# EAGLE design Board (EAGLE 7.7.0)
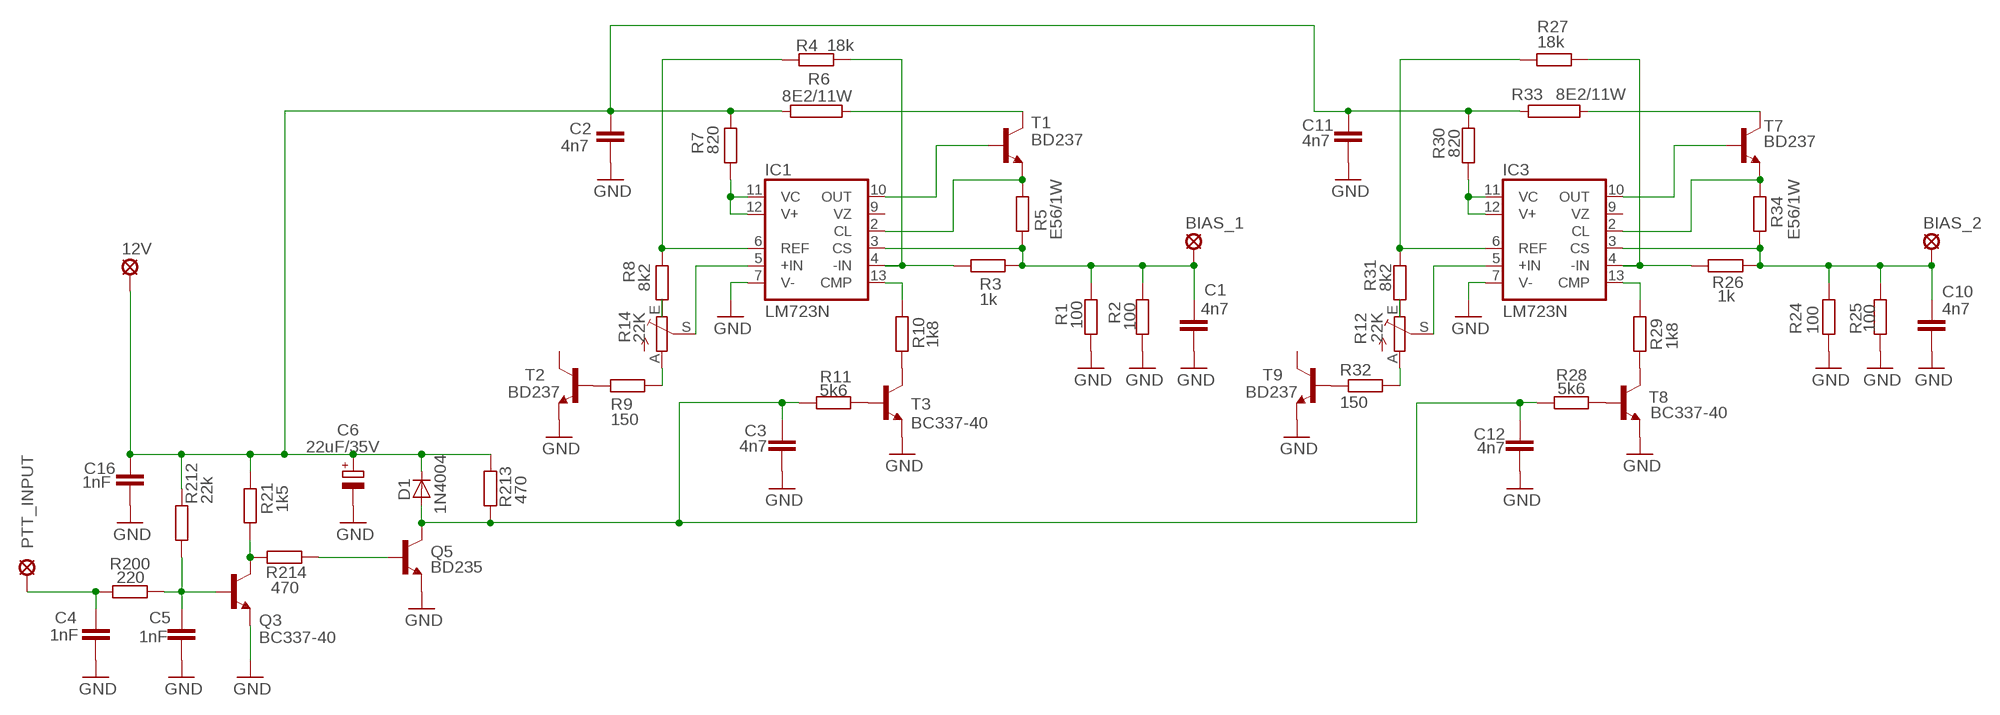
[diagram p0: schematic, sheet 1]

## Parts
12V  MCS10B  [MCS10B]
BIAS_1  MCS10B  [MCS10B]
BIAS_2  MCS10B  [MCS10B]
C1  4n7  C-EU050-024X044  [C050-024X044]
C2  4n7  C-EU050-024X044  [C050-024X044]
C3  4n7  C-EU050-024X044  [C050-024X044]
C4  1nF  C-EU050-024X044  [C050-024X044]
C5  1nF  C-EU050-024X044  [C050-024X044]
C6  22uF/35V  CPOL-EUE5-8.5  [E5-8,5]
C10  4n7  C-EU050-024X044  [C050-024X044]
C11  4n7  C-EU050-024X044  [C050-024X044]
C12  4n7  C-EU050-024X044  [C050-024X044]
C16  1nF  C-EU050-024X044  [C050-024X044]
D1  1N4004  [DO41-10]
IC1  LM723N  [DIL14]
IC3  LM723N  [DIL14]
PTT_INPUT  MCS10B  [MCS10B]
Q3  BC337-40  [TO92]
Q5  BD235  [TO126]
R1  100  R-EU_0207/10  [0207/10]
R2  100  R-EU_0207/10  [0207/10]
R3  1k  R-EU_0207/10  [0207/10]
R4  18k  R-EU_0207/10  [0207/10]
R5  E56/1W  R-EU_0613/15  [P0613/15]
R6  8E2/11W  RKH216-8  [KH216-8]
R7  820  R-EU_0207/10  [0207/10]
R8  8k2  R-EU_0207/10  [0207/10]
R9  150  R-EU_0207/10  [0207/10]
R10  1k8  R-EU_0207/10  [0207/10]
R11  5k6  R-EU_0207/10  [0207/10]
R12  22K  TRIM_EU-B64W  [B64W]
R14  22K  TRIM_EU-B64W  [B64W]
R21  1k5  R-EU_0207/10  [0207/10]
R24  100  R-EU_0207/10  [0207/10]
R25  100  R-EU_0207/10  [0207/10]
R26  1k  R-EU_0207/10  [0207/10]
R27  18k  R-EU_0207/10  [0207/10]
R28  5k6  R-EU_0207/10  [0207/10]
R29  1k8  R-EU_0207/10  [0207/10]
R30  820  R-EU_0207/10  [0207/10]
R31  8k2  R-EU_0207/10  [0207/10]
R32  150  R-EU_0207/10  [0207/10]
R33  8E2/11W  RKH216-8  [KH216-8]
R34  E56/1W  R-EU_0613/15  [P0613/15]
R200  220  R-EU_0207/10  [0207/10]
R212  22k  R-EU_0207/10  [0207/10]
R213  470  R-EU_0207/10  [0207/10]
R214  470  R-EU_0207/10  [0207/10]
T1  BD237  BD235  [TO126]
T2  BD237  BD235  [TO126]
T3  BC337-40  [TO92]
T7  BD237  BD235  [TO126]
T8  BC337-40  [TO92]
T9  BD237  BD235  [TO126]

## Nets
N$1: R29.2 T8.3(C)
N$2: IC1.13(CMP) R10.1
N$3: C3.1 C12.1 D1.A Q5.2(C) R11.1 R28.1 R213.1
N$4: R11.2 T3.2(B)
N$5: IC1.11(VC) IC1.12(V+) R7.1
N$6: C4.1 PTT_INPUT.MP R200.1
N$7: R6.2 T1.2(C)
N$8: IC1.10(OUT) T1.3(B)
N$9: IC1.2(CL) R5.2 T1.1(E)
N$10: BIAS_1.MP C1.1 IC1.3(CS) R1.2 R2.2 R3.2 R5.1
N$11: IC1.4(-IN) R3.1 R4.2
N$12: IC1.5(+IN) R14.S
N$13: IC1.6(REF) R4.1 R8.2
N$14: R8.1 R14.E
N$15: R9.2 R14.A
N$16: R9.1 T2.3(B)
N$17: C1.2 C2.2 C3.2 C4.2 C5.2 C6.- C10.2 C11.2 C12.2 C16.2 IC1.7(V-) IC3.7(V-) Q3.1(E) Q5.1(E) R1.1 R2.1 R24.1 R25.1 T2.1(E) T3.1(E) T8.1(E) T9.1(E) ; supply symbol labelled GND
N$18: 12V.MP C2.1 C6.+ C11.1 C16.1 D1.C R6.1 R7.2 R21.2 R30.2 R33.1 R212.2 R213.2
N$20: R10.2 T3.3(C)
N$22: C5.1 Q3.2(B) R200.2 R212.1
N$34: IC3.13(CMP) R29.1
N$35: R28.2 T8.2(B)
N$37: IC3.11(VC) IC3.12(V+) R30.1
N$38: Q3.3(C) R21.1 R214.1
N$39: R33.2 T7.2(C)
N$40: IC3.10(OUT) T7.3(B)
N$41: IC3.2(CL) R34.2 T7.1(E)
N$42: BIAS_2.MP C10.1 IC3.3(CS) R24.2 R25.2 R26.2 R34.1
N$43: IC3.4(-IN) R26.1 R27.2
N$44: IC3.5(+IN) R12.S
N$45: IC3.6(REF) R27.1 R31.2
N$46: R12.E R31.1
N$47: R12.A R32.2
N$48: R32.1 T9.3(B)
N$54: Q5.3(B) R214.2
Unconnected: IC1.9(VZ) IC3.9(VZ) T2.2(C) T9.2(C)

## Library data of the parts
12V BIAS_1 BIAS_2 PTT_INPUT = solpad:MCS10B: SOLDER PAD
C1-C5 C10-C12 C16 = rcl:C-EU: CAPACITOR, European symbol
C6 = rcl:CPOL-EU: POLARIZED CAPACITOR, European symbol
D1 = diode:1N4004: DIODE
IC1 IC3 = linear:*723: Positive VOLTAGE REGULATOR
Q3 T3 T8 = transistor-npn:BC337*: NPN Transistor
Q5 T1 T2 T7 T9 = transistor-npn:BD235*: NPN Transistor
R1-R5 R7-R11 R21 R24-R32 R34 R200 R212-R214 = rcl:R-EU_: RESISTOR, European symbol
R6 R33 = resistor-power:R: Power Resitor
R12 R14 = pot:TRIM_EU-: POTENTIOMETER

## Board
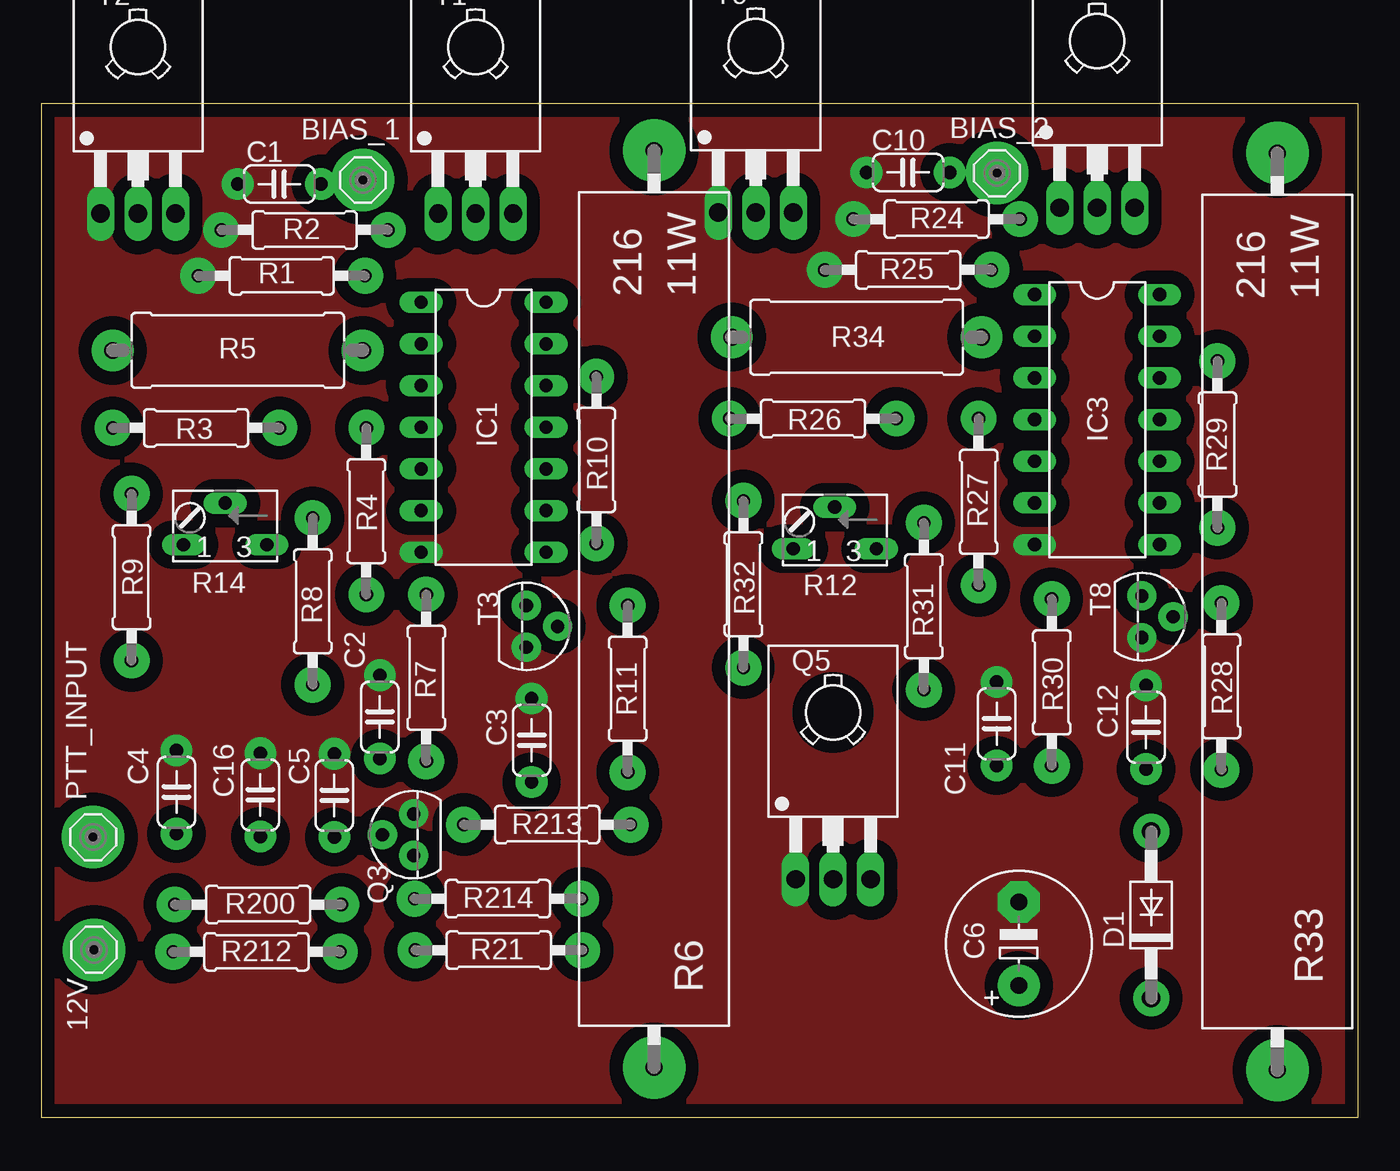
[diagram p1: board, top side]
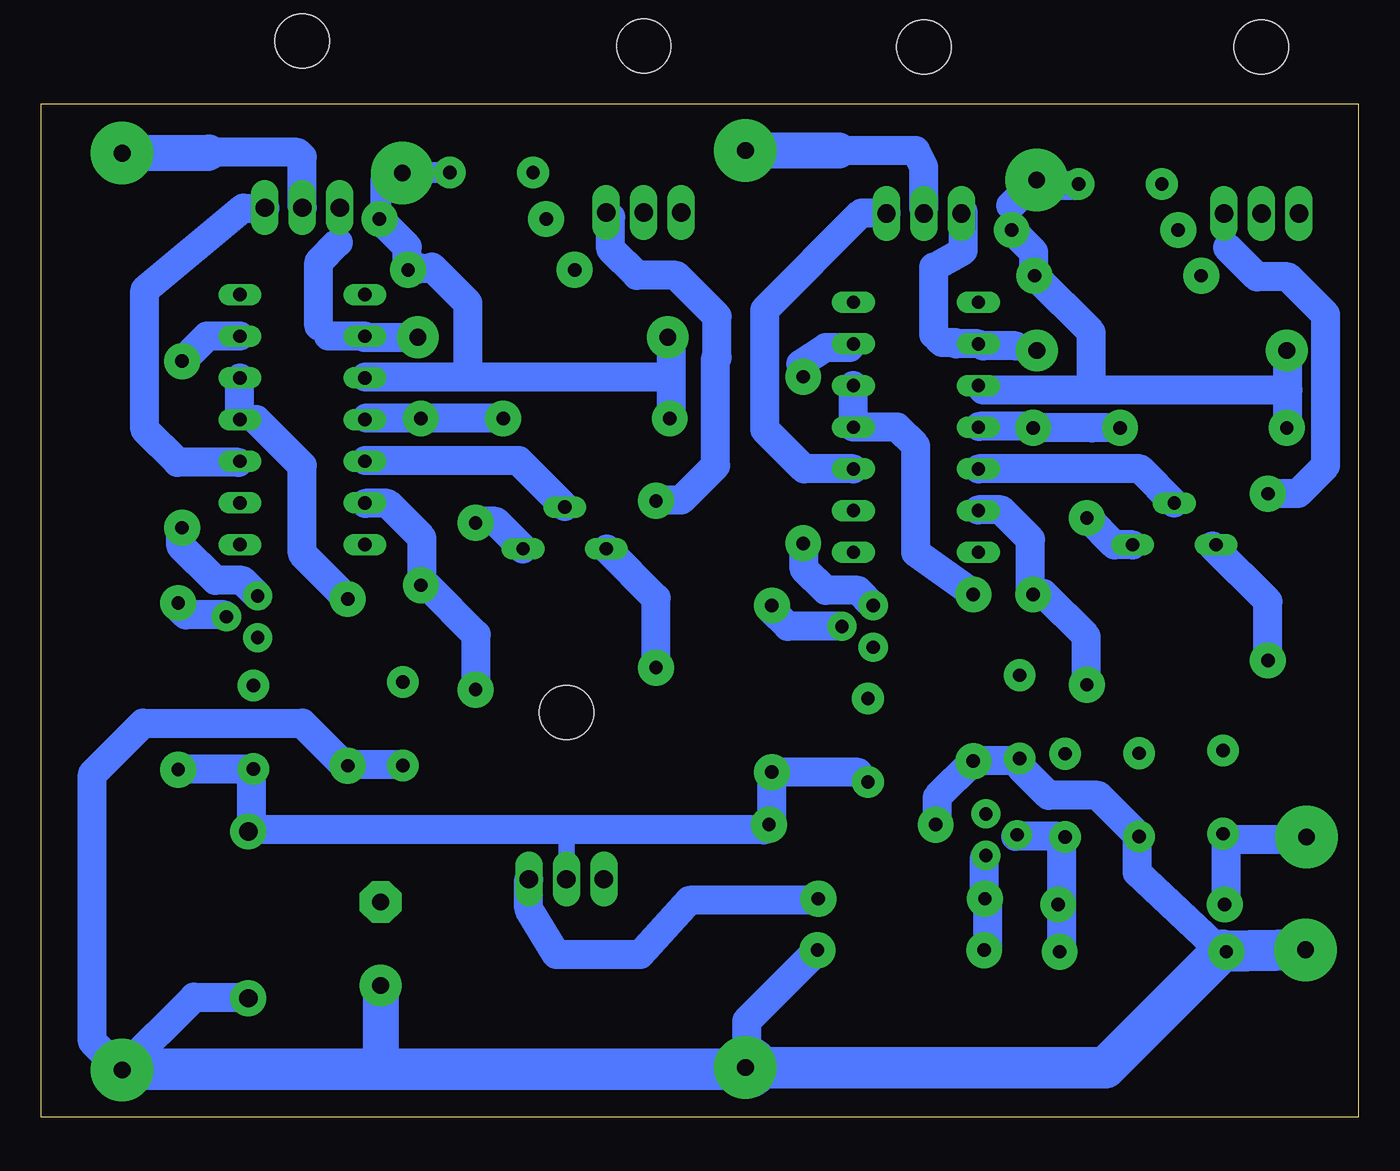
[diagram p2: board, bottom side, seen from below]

Size 80.33 x 61.8 mm. Coordinates in mm from the lower left corner, seen from the top.
Outline: 0,0 80.33,0 80.33,61.8 0,61.8 0,0
Copper layers (1*16): Top 0.035mm / dielectric 1.5mm / Bottom 0.035mm
Design rules "default": minimum track width 10mil, minimum drill 24mil, track to track 8mil, track to pad 8mil, pad to pad 8mil, via to via 8mil, smd to smd 8mil, copper to edge 20mil, drill to drill 8mil, minimum pad ring 10mil, minimum via ring 8mil, stop-mask expansion 4mil, vias tented up to drill 0mil, thermal gap 10mil

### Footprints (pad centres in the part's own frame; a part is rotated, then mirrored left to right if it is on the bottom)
MCS10B = drill 1.016 pad 3.81: MP 0,0
C050-024X044 = drill 0.813 pad 1.93: 1 -2.54,0; 2 2.54,0
E5-8,5 = drill 1.016 pad 2.54: + -2.54,0 | drill 1.016 pad 2.54 octagon: - 2.54,0
DO41-10 = drill 1.118 pad 2.184: A 5.08,0; C -5.08,0
DIL14 = drill 0.813 long: 1 -7.62,-3.81; 2 -5.08,-3.81; 3 -2.54,-3.81; 4 0,-3.81; 5 2.54,-3.81; 6 5.08,-3.81; 7 7.62,-3.81; 8 7.62,3.81; 9 5.08,3.81; 10 2.54,3.81; 11 0,3.81; 12 -2.54,3.81; 13 -5.08,3.81; 14 -7.62,3.81
TO92 = drill 0.813 pad 1.778: 1 1.27,0; 2 0,1.905; 3 -1.27,0
TO126 = drill 1.118 long: 1 -2.286,-5.08; 2 0,-5.08; 3 2.286,-5.08 | hole 3.302: 0,5.08
0207/10 = drill 0.813 pad 2.184: 1 -5.08,0; 2 5.08,0
P0613/15 = drill 1.016 pad 2.54: 1 -7.62,0; 2 7.62,0
KH216-8 = drill 1.016 pad 3.81: 1 -27.94,0; 2 27.94,0
B64W = drill 0.813 long: A 2.54,0; E -2.54,0; S 0,-2.54

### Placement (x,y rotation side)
12V  3.23,10.22 0 top
BIAS_1  19.63,57.14 0 top
BIAS_2  58.29,57.56 0 top
C1  14.53,56.89 180 top
C2  20.66,24.41 90 top
C3  29.91,22.99 90 top
C4  8.26,19.83 90 top
C5  17.88,19.63 90 top
C6  59.62,10.59 90 top
C10  52.87,57.6 180 top
C11  58.27,24 90 top
C12  67.37,23.78 90 top
C16  13.37,19.66 90 top
D1  67.69,12.35 90 top
IC1  26.99,42.07 270 top
IC3  64.4,42.54 270 top
PTT_INPUT  3.18,17.09 0 top
Q3  22.71,17.24 90 top
Q5  48.29,19.6 0 top
R1  14.67,51.3 0 top
R2  16.07,54.1 0 top
R3  9.45,42.03 180 top
R4  19.83,36.95 90 top
R5  11.99,46.75 0 top
R6  37.38,30.99 90 top
R7  23.49,26.8 270 top
R8  16.56,31.46 270 top
R9  5.52,32.94 270 top
R10  33.86,40.07 270 top
R11  35.77,26.13 90 top
R12  48.4,34.66 180 top
R14  11.23,34.9 180 top
R21  27.91,10.2 0 top
R24  54.61,54.76 0 top
R25  52.87,51.66 0 top
R26  47.07,42.6 180 top
R27  57.17,37.52 90 top
R28  71.97,26.28 90 top
R29  71.73,41.02 270 top
R30  61.63,26.52 270 top
R31  53.83,31.16 270 top
R32  42.83,32.5 270 top
R33  75.38,30.83 90 top
R34  49.73,47.56 0 top
R200  13.24,12.98 0 top
R212  13.14,10.1 180 top
R213  30.86,17.85 180 top
R214  27.86,13.33 0 top
T1  26.49,60.17 0 top
T2  5.92,60.17 0 top
T3  29.59,29.93 270 top
T7  64.4,60.53 0 top
T8  67.12,30.52 270 top
T9  43.58,60.23 0 top

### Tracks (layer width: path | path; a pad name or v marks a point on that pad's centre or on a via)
N$1
  Bottom 1.016: 71.8,35.87 R29.2
  Bottom 1.778: T8.3 68.06,32.73 69.7,32.73 71.8,34.83 71.8,35.87
N$2
  Bottom 1.27: IC1.13 31.02,46.93 | R10.1 33.58,45.43 34,45.43 34,45.93
  Bottom 1.778: 31.02,46.93 32.5,46.93 34,45.93
N$3
  Bottom 0.406: R28.1 71.93,21.2 71.89,21.24
  Bottom 1.016: D1.A 67.7,17.53 67.5,17.73 | 36.27,17.53 R213.1 35.82,17.73 35.8,17.73 | Q5.2 48.3,17.53 | 35.8,21.03 35.79,21.03 R11.1 35.8,21.02 | C3.1 30.49,21.03
  Bottom 1.27: 67.5,21.24 C12.1
  Bottom 1.778: 71.89,21.24 67.5,21.24 67.5,17.73 | 36.27,17.53 48.3,17.53 67.7,17.53 | 30.49,21.03 35.79,21.03 | 35.8,21.02 35.8,17.73
N$4
  Bottom 1.016: T3.2 | 35.8,31.24 35.8,31.33 | 35.8,31.24 R11.2 | 35.8,30.93 35.8,31.24
  Bottom 1.778: T3.2 34.8,29.93 35.8,30.93
N$5
  Bottom 0.406: IC1.11 30.8,42.13 30.5,42.43 30.8,42.73 | R7.1 23.49,31.92
  Bottom 1.778: 30.8,42.73 IC1.12 | IC1.11 28.14,42.07 27,40.93 27,34.43 23.49,31.92
N$6
  Bottom 0.61: 3.34,16.93 PTT_INPUT.MP | 8.1,12.93 8.1,13.12 R200.1 | 8.1,16.93 C4.1
  Bottom 1.778: 3.34,16.93 8.1,16.93 8.1,13.12
N$7
  Bottom 0.406: 26.5,55.43 26.49,55.43 T1.2
  Bottom 1.778: 26.5,55.43 26.5,57.93 27,58.93 31.7,58.93
  Bottom 1.93: 31.7,58.93 32,58.93
  Bottom 2.184: R6.2 31.7,58.93
N$8
  Bottom 1.016: IC1.10 | 28.8,55.13 28.8,55.11 T1.3
  Bottom 1.778: IC1.10 33.8,39.53 36.2,41.93 36.2,49.23 30.3,55.13 28.8,55.13
N$9
  Bottom 1.016: IC1.2 23.1,47.23 22.9,47.03 | 20.7,47.03 20.9,47.03 19.89,47.03 R5.2 | 24.52,47.15 24.6,47.23 | 24.1,55.23 24.1,55.2 T1.1
  Bottom 1.778: 20.9,47.03 22.9,47.03 | IC1.2 24.52,47.15 | 24.6,47.23 25.4,47.23 25.9,47.73 25.9,51.83 24.1,52.83 24.1,55.2
N$10
  Bottom 1.016: BIAS_1.MP 19.61,57.13 19.4,57.13 19.1,56.83 | 17.1,56.83 17.1,56.86 C1.1 | R2.2 21.2,54.14 21.2,55.57 | 4.3,46.73 4.35,46.73 R5.1 | R3.2 4.3,42.11 | 22.89,44.33 IC1.3 | 19.8,51.33 19.78,51.33 R1.2
  Bottom 1.778: 19.1,56.83 17.1,56.83 | 21.2,55.57 BIAS_1.MP | 4.3,42.11 4.3,44.33 | 4.3,44.33 4.3,46.73 | 4.3,44.33 16.3,44.33 | 16.3,44.33 22.89,44.33 | R2.2 19.8,52.74 19.8,51.33 | R1.2 16.3,47.85 16.3,44.33
N$11
  Bottom 1.016: R4.2 19.93,42.13 | 23.12,42.13 IC1.4
  Bottom 1.778: R3.1 16.24,42.03 R4.2 | 19.93,42.13 23.12,42.13
N$12
  Bottom 1.016: IC1.5
  Bottom 1.778: R14.S 13.32,39.53 IC1.5
N$13
  Bottom 1.016: R8.2 16.6,26.42 | 19.2,31.93 19.8,31.93 19.8,31.91 R4.1 20,32.04 | 23.2,37.03 23.2,37.01 IC1.6
  Bottom 1.778: 16.6,26.42 16.6,29.33 19.2,31.93 | 20,32.04 20,35.23 21.8,37.03 23.2,37.03
N$14
  Bottom 0.406: R8.1 16.66,37.09
  Bottom 1.016: 16.51,36.54 R8.1
  Bottom 1.778: R14.E 14.87,34.9 16.51,36.54
N$15
  Bottom 1.27: 8.9,34.83 8.82,34.9 R14.A
  Bottom 1.778: R9.2 5.52,31.46 8.9,34.83
N$16
  Bottom 1.016: 5.51,38.03 R9.1 | T2.3 8,54.88 8,53.03
  Bottom 1.778: 5.51,38.03 3.7,38.03 2,39.73 2,48.93 4.3,51.23 6.2,51.23 8,53.03
N$17
  pour Top (isolate 0.813, no thermals): 0.3,61.13 0.3,0.23 79.7,0.23 79.7,61.33
N$18
  Bottom 0.406: 8.4,10.13 10.19,7.33 R212.2
  Bottom 0.61: 8.46,10.13 R212.2 | 12V.MP 3.24,10.23
  Bottom 1.016: 58.34,21.53 C11.1 | 61.9,21.53 61.7,21.33 | 75.4,2.93 75.4,2.91 R33.1 75.4,2.87 | 75.4,2.93 75.5,2.93 | 37.3,2.93 37.3,3.05 | 67.75,7.33 D1.C | 75.4,2.87 75.4,2.83 | 75.4,2.93 75.4,2.87 | 59.6,2.93 59.6,2.53 | 59.6,8.03 C6.+
  Bottom 1.27: 13.5,16.75 C16.1 | R30.2 61.51,21.44 61.5,21.43 61.47,21.46 C11.1
  Bottom 1.778: 13.5,16.75 13.5,14.93 8.4,10.13 | 58.34,21.53 61.9,21.53 64.4,24.03 74.1,24.03 77.2,20.93 77.2,4.63 75.5,2.93 | 67.75,7.33 71,7.33 75.4,2.93 | R21.2 37.3,5.89 37.3,4.63 | 37.3,4.63 37.3,3.73 | C16.1 15.88,19.63 18.9,19.63 20.6,21.33 20.6,21.93 C2.1 20.8,21.73 R7.2 | R7.2 | R7.2 25.7,19.51 25.7,17.93 25.71,17.93 R213.2 | R6.1 37.3,3.13 37.3,4.63
  Bottom 1.93: R212.2 8.27,10.2
  Bottom 2.184: 59.6,2.93 59.6,8.03
  Bottom 2.54: 3.24,10.23 8.46,10.13 | 37.5,2.93 37.3,2.93 | 37.5,2.93 59.6,2.93 75.4,2.93 | 37.5,2.93 37.5,3.03 15.44,3.03 8.27,10.2
  Bottom 3.81: 37.3,3.05 R6.1
N$20
  Bottom 1.016: 33.8,35.03 33.82,35.03 R10.2
  Bottom 1.778: T3.3 30.52,32.13 32.5,32.13 33.8,33.43 33.8,35.03
N$22
  Bottom 0.406: 21,17.13 20.92,17.13 Q3.2 | 18.1,17.03 18.3,17.13 | 18.6,13.43 18.57,13.43 R200.2 | 18.1,13.23 18.6,13.43 | 18.6,13.43 18.8,13.43
  Bottom 0.61: R212.1 18.1,10.52 | 18.1,17.03 18.04,16.93 C5.1
  Bottom 1.778: 18.1,10.52 18.1,13.23 18.1,17.03 | 18.3,17.13 20.92,17.13
N$34
  Bottom 1.778: IC3.13 70.21,47.62 R29.1
N$35
  Bottom 1.016: T8.2 69.13,30.63 | R28.2 72,31.33 72,31.13
  Bottom 1.778: 69.13,30.63 71.5,30.63 72,31.13
N$37
  Bottom 0.406: IC3.11 68.21,42.62 68.1,42.73 68.15,42.78 68.21,42.84
  Bottom 1.016: 68.15,42.78 68.4,42.53 67.2,42.53
  Bottom 1.778: 68.21,42.84 IC3.12 | R30.1 64.4,34.37 64.4,39.73 67.2,42.53
N$38
  Bottom 0.406: 22.8,13.23 22.8,13.31 R214.1 22.6,13.16 | 22.8,15.88 Q3.3 | R21.1 22.6,10.43
  Bottom 1.778: 22.8,13.31 22.8,15.88 | 22.6,10.43 22.6,13.16
N$39
  Bottom 1.778: T7.2 64.4,58.53 64.7,58.83 70.1,58.83 70.2,58.73 70.2,58.77
  Bottom 2.184: R33.2 70.2,58.77 70.16,58.77 70.1,58.83
N$40
  Bottom 0.406: T7.3
  Bottom 1.27: IC3.10 68.28,39.93 | 66.5,55.43 66.66,55.43 T7.3
  Bottom 1.778: 68.28,39.93 72,39.93 74,41.93 74,50.43 68,55.43 66.66,55.43
N$41
  Bottom 1.016: 60.6,47.53 IC3.2 | R34.2 57.38,47.53 | 62.8,47.63 63.4,48.23 | T7.1 62.2,55.36 62.2,53.33
  Bottom 1.778: 57.38,47.53 60.6,47.53 | IC3.2 62.8,47.63 | 63.4,48.23 63.4,52.13 62.2,53.33
N$42
  Bottom 0.406: 59.6,57.13 59.15,57.58 59.13,57.6 | 59.69,54.84 59.7,54.83 | R24.2 59.69,54.84 | 59.69,54.84 59.6,54.93
  Bottom 1.016: R26.2 41.9,42.69 | 41.9,47.35 R34.1 | 60.54,45.13 IC3.3 | 57.6,51.71 R25.2 57.38,51.83 | 54.3,45.13 54.3,45.03 | 59.15,57.58 59.2,57.63 58.36,57.63 BIAS_2.MP
  Bottom 1.27: 59.13,57.6 C10.1 | 59.6,54.93 59.6,57.13
  Bottom 1.778: 41.9,42.69 41.9,45.13 | 41.9,45.13 41.9,47.35 | 41.9,45.13 54.3,45.13 | 54.3,45.13 60.54,45.13 | 54.3,45.13 54.3,49.63 56.5,51.83 56.6,51.73 57.28,51.73 57.38,51.83 | R25.2 58,51.71 58,53.07 R24.2
N$43
  Bottom 1.016: 57.2,42.63 57.3,42.63 | 57.2,42.63 R27.2 | R26.1 52.18,42.63 | 56.9,42.63 57.2,42.63 | 60.5,42.63 IC3.4
  Bottom 1.778: 52.18,42.63 56.9,42.63 60.5,42.63
N$44
  Bottom 1.016: 60.56,40.03 IC3.5 | 48.3,37.23 48.37,37.23 | 48.37,37.23 R12.S | 48.37,37.23 48.4,37.23
  Bottom 1.778: 60.56,40.03 51.2,40.03 48.4,37.23
N$45
  Bottom 1.016: R31.2 53.8,26.11 | 56.8,32.43 R27.1 57.1,32.51 | 60.56,37.43 IC3.6
  Bottom 1.778: 53.8,26.11 53.8,29.43 56.8,32.43 | 57.1,32.51 57.1,35.33 59.2,37.43 60.56,37.43
N$46
  Bottom 1.016: 53.8,36.33 53.8,36.27 R31.1
  Bottom 1.778: R12.E 52.61,36.33 53.8,36.33
N$47
  Bottom 0.406: 45.83,34.66 R12.A
  Bottom 1.778: R32.2 42.83,31.66 45.83,34.66
N$48
  Bottom 1.016: 42.78,37.63 R32.1 | 39.1,46.73 39.2,46.73 39.2,46.33 39.1,46.33 | 45.6,54.88 T9.3
  Bottom 1.778: 42.78,37.63 41.3,37.63 39.2,39.73 39.2,46.33 | 45.6,54.88 45.6,52.93 44,51.33 41.6,51.33 39.1,48.83 39.1,46.33
N$54
  Bottom 0.406: R214.2 33.04,13.23 | 50.6,14.51 Q5.3
  Bottom 1.778: 33.04,13.23 40.8,13.23 43.8,9.93 48.9,9.93 50.6,12.73 50.6,14.51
